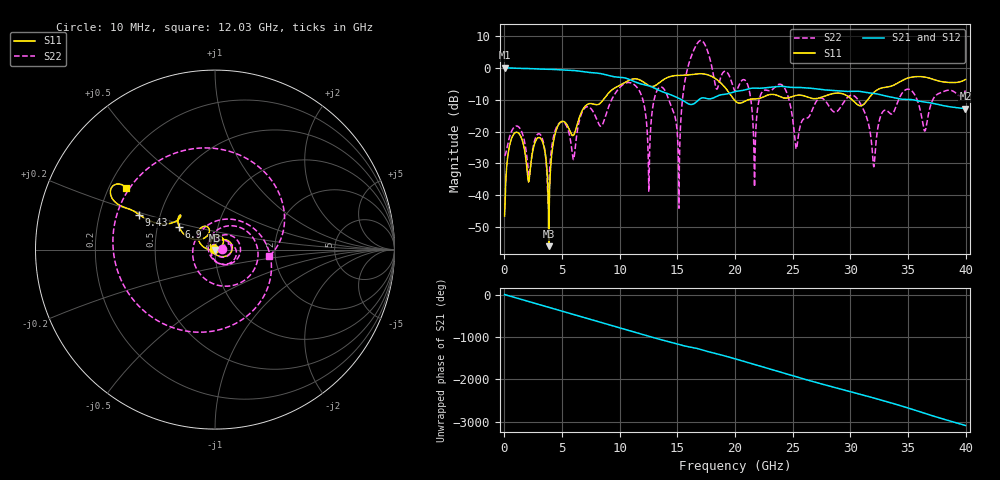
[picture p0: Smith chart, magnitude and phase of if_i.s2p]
!Keysight Technologies,N5245B,MY57181346,A.12.70.07
!Automatic Fixture Removal (AFR)
!Date: Wednesday, November 07, 2018 11:44:22 AM
!S2P File: Measurements: S11,S21,S12,S22:
# MHz S  RI  R 50
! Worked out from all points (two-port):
!   3999 points, 10 MHz to 39.99 GHz, reference 50 ohm
!   highest |S21| = -0.01 dB at 10 MHz (marker M1); lowest = -12.9 dB at 39.99 GHz (marker M2)
!   |S21| within 3 dB of the highest: start of sweep to 10.13 GHz
!   lowest |S11| = -55.9 dB at 3.84 GHz (marker M3), VSWR 1.00, Z = 50.1 - j0.139 ohm
!   |S11| at or under -10 dB: start of sweep to 8.577 GHz; 19.92 GHz to 21.18 GHz (1.256 GHz wide, 6.11 % of centre); 30.15 GHz to 31.51 GHz (1.365 GHz wide, 4.43 % of centre)
!   |S22| runs from -44.0 to 8.6 dB; largest |S21 - S12| = 1.5e-15
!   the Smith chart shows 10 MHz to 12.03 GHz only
!   S11 on the Smith chart (normalised r, x): 10 MHz: 0.99, +0.00; 6.9 GHz: 0.65, +0.17; 9.43 GHz: 0.38, +0.19; 12.03 GHz: 0.27, +0.29
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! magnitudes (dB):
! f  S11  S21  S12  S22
! 10 MHz  -46.5  0.0  0.0  -27.6
! 1 GHz  -20.2  -0.2  -0.2  -18.3
! 3.84 GHz  -55.9  -0.5  -0.5  -38.4
! 4.6 GHz  -18.5  -0.6  -0.6  -18.0
! 6.68 GHz  -13.9  -1.2  -1.2  -14.4
! 6.9 GHz  -12.5  -1.3  -1.3  -12.9
! 9.43 GHz  -6.7  -2.8  -2.8  -9.1
! 12.03 GHz  -4.4  -5.2  -5.2  -10.4
! 12.53 GHz  -5.6  -5.7  -5.7  -38.8
! 13.34 GHz  -4.9  -7.0  -7.0  -6.5
! 15.09 GHz  -2.4  -9.5  -9.5  -29.3
! 16.84 GHz  -1.9  -10.1  -10.1  8.2
! 20 GHz  -10.3  -7.5  -7.5  -7.3
! 21.06 GHz  -10.2  -6.7  -6.7  -5.0
! 21.7 GHz  -9.8  -6.4  -6.4  -36.4
! 22.52 GHz  -9.1  -6.3  -6.3  -7.1
! 25.33 GHz  -8.7  -6.2  -6.2  -25.4
! 26.67 GHz  -9.6  -6.5  -6.5  -13.5
! 30.4 GHz  -10.9  -7.4  -7.4  -9.0
! 32.04 GHz  -7.8  -8.0  -8.0  -31.0
! 33.33 GHz  -6.0  -9.1  -9.1  -13.9
! 39.99 GHz  -3.7  -12.9  -12.9  -7.1
